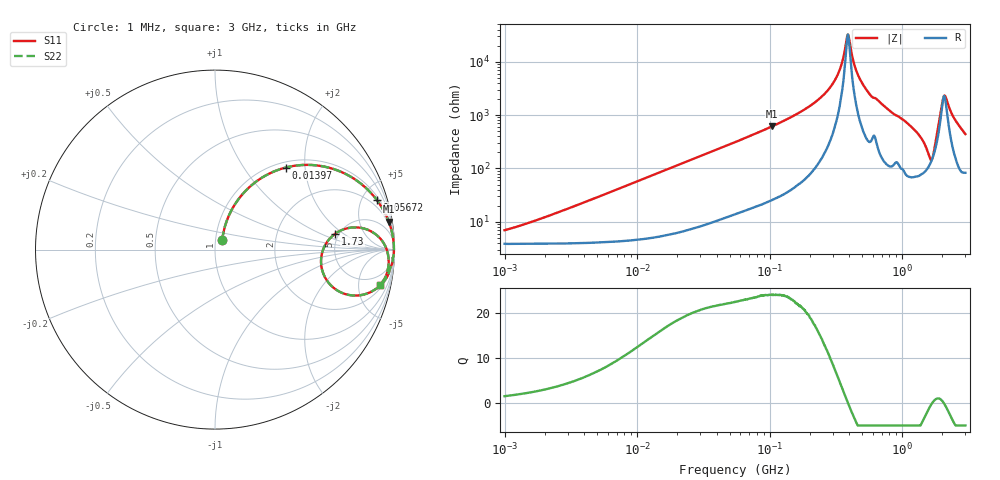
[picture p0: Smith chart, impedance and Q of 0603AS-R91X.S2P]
!s-Parameter Generated by FASTRON Sdn. Bhd.
!FASTRON P/N : 0603AS-R91X
!Keysight Technologies: E4991B_MY54100416_A.01.15
!Date created: Tue Oct 17 15:54:33 2023
!Version  : Rev01 Tue Oct 17 15:54:33 2023
!Data & Calibration Information:
!Freq	S11	S21	S12	S22
!PortZ  Port1:50+j0  Port2:50+j0
!When reading reference impedance value at option line is always used.
! Remarks : This data is being provided solely for informational purposes.
# Hz S dB R 50
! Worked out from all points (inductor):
!   1601 points, 1 MHz to 3 GHz, reference 50 ohm
!   read as one part in series: L = 913 nH near 2.045 MHz
!   highest Q = 24 at 104.4 MHz (marker M1), where L = 936 nH
!   self-resonance near 389.5 MHz
!   S11 on the Smith chart (normalised r, x): 1 MHz: 1.08, +0.12; 13.97 MHz: 1.10, +1.59; 56.72 MHz: 1.29, +6.42; 1.73 GHz: 4.65, +1.52; 3 GHz: 2.66, -8.62
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1000000  -23.49 52.9  -0.34 -3.2  -0.34 -3.2  -23.49 52.9
3804036  -13.62 67.8  -0.53 -11.8  -0.53 -11.8  -13.62 67.8
1.397259e7  -4.38 49.2  -2.40 -37.1  -2.40 -37.1  -4.38 49.2
1.447069e7  -4.20 48.3  -2.51 -38.0  -2.51 -38.0  -4.20 48.3
5.477226e7  -0.54 17.6  -10.37 -69.8  -10.37 -69.8  -0.54 17.6
5.672481e7  -0.51 17.0  -10.65 -70.4  -10.65 -70.4  -0.51 17.0
1.044488e8  -0.17 9.2  -15.95 -78.4  -15.95 -78.4  -0.17 9.2
2.083556e8  -0.05 3.6  -23.97 -83.2  -23.97 -83.2  -0.05 3.6
3.124888e8  -0.03 1.2  -33.31 -80.8  -33.31 -80.8  -0.03 1.2
3.453811e8  -0.03 0.7  -38.38 -75.1  -38.38 -75.1  -0.03 0.7
3.894533e8  -0.03 0.0  -50.21 -1.5  -50.21 -1.5  -0.03 0.0
4.435663e8  -0.03 -0.7  -37.63 74.8  -37.63 74.8  -0.03 -0.7
5.001674e8  -0.03 -1.4  -31.88 80.4  -31.88 80.4  -0.03 -1.4
7.925923e8  -0.09 -4.5  -21.98 80.3  -21.98 80.3  -0.09 -4.5
1.268618e9  -0.41 -11.0  -14.32 70.9  -14.32 70.9  -0.41 -11.0
1.519029e9  -1.70 -18.1  -9.46 49.6  -9.46 49.6  -1.70 -18.1
1.637435e9  -4.19 -12.4  -7.56 18.4  -7.56 18.4  -4.19 -12.4
1.730092e9  -3.40 7.5  -9.32 -15.1  -9.32 -15.1  -3.40 7.5
1.883708e9  -0.93 5.5  -17.33 -39.1  -17.33 -39.1  -0.93 5.5
2.092429e9  -0.35 -0.8  -27.66 18.4  -27.66 18.4  -0.35 -0.8
2.480502e9  -0.27 -6.4  -18.88 71.3  -18.88 71.3  -0.27 -6.4
3e9  -0.56 -12.1  -13.41 67.0  -13.41 67.0  -0.56 -12.1
